PROGRAM MAIN
VAR
	MisMotorAxis1 : MIS_Ctrl; //Instance of motor to control
	ProfilePositioni: MIS_ProfilePosition; //instandce of the profilePositioning functione block
	ProfileHomingi: MIS_ProfileHoming; //Instance of the Homing profile function block
	MISenableMotori: MIS_EnableMotor;
	ChangeMode: MIS_ChangeDSP402Mode;
	ProfileVelocityi: MIS_ProfileVelocity;

	//Test variables
	bModeactive: BOOL;
	eCommandLocal: ECOMMAND;
	diTargetVelocity : DINT := 75;
	rPos1 : REAL := 10;
	rpos2 : REAL := -10; 
END_VAR

VAR_INPUT
	iState : INT ; //State of main function
END_VAR

//wNodeID CANopen node adress of motor
//ADSNetID Adress of the CANopen adapter. Get the ADS net id from the CANopen master adapter, In this example is used an EL6751 adapter
//lrUnitConversion Counts pr unit. This sample uses counts Pr revolution as Convertion factor.
MisMotorAxis1(wNode := 5,ADSNetID := '5.80.217.236.3.1',lrUnitConversion := 409600);


CASE iState OF
0:
	//Reset function blocks
	ProfilePositioni(eCmd := eCommand.Reset,stMisMotorLocal := MisMotorAxis1.stMisMotori);
	ProfileHomingi(eCmd := eCommand.Reset,stMisMotorLocal := MisMotorAxis1.stMisMotori);
	ProfileVelocityi(eCmd := eCommand.Reset,stMisMotorLocal := MisMotorAxis1.stMisMotori);
	ChangeMode(eCmd := eCommand.Reset,stMisMotorLocal := MisMotorAxis1.stMisMotori);

	
	// Set iState to a value to try the function block.
	//
	// 10 Profile postition mode
	// 50 Velocity mode
	// 70 Homing mode
	// 100 Enable motor
	// 110 Disable motor 
	

/////////////////////////////////////////////////////////////////////////////////////////////////////////////////////////////	
10: //Test Profile position
	ChangeMode(eCmd := eCommand.Run,siModeOfOperation := 1,stMisMotorLocal := MisMotorAxis1.stMisMotori);
	IF ChangeMode.eStat = eStatus.Done THEN
		ChangeMode(eCmd := eCommand.Reset,stMisMotorLocal := MisMotorAxis1.stMisMotori);
		bModeactive := TRUE;
		iState := iState + 1;
		eCommandLocal := eCommand.Run;		
	END_IF
11:
	ProfilePositioni(eCmd := eCommand.Reset,rVelocityRpm := 100, rAccellRpms := 100, lrTargetPos := rPos1,stMisMotorLocal := MisMotorAxis1.stMisMotori);
	//iState := 20;  //Sequntial profiles 
	iState := 30; //Overlapping profiles
	
		
//Alternating between 2 positions. Waiting for position reached before next profile prepared
//This allow aborting with quickstop by appliyng the Command stop
20: //Alternate between 2 positions. Wait for position reached 
	IF NOT bModeactive THEN eCommandLocal := eCommand.Stop; END_IF; //Force stop
	ProfilePositioni(eCmd := eCommandLocal,stMisMotorLocal := MisMotorAxis1.stMisMotori);
	IF ProfilePositioni.eStat = eStatus.Done THEN //Wait for position reached
		iState := iState + 1;
	END_IF
	
21:
	IF ProfilePositioni.lrTargetPos <> rPos1 THEN 
		ProfilePositioni(eCmd := eCommand.Reset,rVelocityRpm := 100, rAccellRpms := 100, lrTargetPos := rPos1,stMisMotorLocal := MisMotorAxis1.stMisMotori);
	ELSE
		ProfilePositioni(eCmd := eCommand.Reset,rVelocityRpm := 200, rAccellRpms := 50, lrTargetPos := rPos2,stMisMotorLocal := MisMotorAxis1.stMisMotori);
	END_IF
	iState := iState + 1;

22:	
	IF bModeactive THEN
		iState := 20;
	END_IF;
	

//Laternating between positions. Next position prepared before previus completed.
//Use the bChangeEmidiatly if new Targetdata should be used before position is reached
30:
	IF NOT bModeactive THEN eCommandLocal := eCommand.Stop; END_IF; //Force stop
	ProfilePositioni(eCmd := eCommandLocal,stMisMotorLocal := MisMotorAxis1.stMisMotori);
	IF ProfilePositioni.eStat = eStatus.CmdOk THEN //Wait for command completed
		iState := iState + 1;
	END_IF
	
31: //Preare next commands
	IF ProfilePositioni.lrTargetPos <> rPos1 THEN 
		ProfilePositioni(eCmd := eCommand.Reset,rVelocityRpm := 100, rAccellRpms := 100, lrTargetPos := rPos1,stMisMotorLocal := MisMotorAxis1.stMisMotori);
	ELSE
		ProfilePositioni(eCmd := eCommand.Reset,rVelocityRpm := 200, rAccellRpms := 50, lrTargetPos := rPos2,stMisMotorLocal := MisMotorAxis1.stMisMotori);
	END_IF
	iState := iState + 1;

32:	
	IF bModeactive THEN
		iState := 30;
	END_IF;
	
	



/////////////////////////////////////////////////////////////////////////////////////////////////////////////////////////////
50: //test profile velocity mode 
	ChangeMode(eCmd := eCommand.Run,siModeOfOperation := 3,stMisMotorLocal := MisMotorAxis1.stMisMotori);
	IF ChangeMode.eStat = eStatus.Done THEN
		ChangeMode(eCmd := eCommand.Reset,stMisMotorLocal := MisMotorAxis1.stMisMotori);
		iState := iState + 1;
	END_IF
	
51:
	ProfileVelocityi(eCmd := eCommand.Run,rVelocityRpm := ANY_TO_REAL(diTargetVelocity),rAccellRpms := 125,stMisMotorLocal := MisMotorAxis1.stMisMotori);
	
		
	
/////////////////////////////////////////////////////////////////////////////////////////////////////////////////////////////
70: //Test profile homing mode
	ChangeMode(eCmd := eCommand.Run,siModeOfOperation := 6,stMisMotorLocal := MisMotorAxis1.stMisMotori);
	IF ChangeMode.eStat = eStatus.Done THEN
		ChangeMode(eCmd := eCommand.Reset,stMisMotorLocal := MisMotorAxis1.stMisMotori);
		iState := iState + 1;
	END_IF

71:
	ProfileHomingi(eCmd := eCommand.Run,iHomingMode := 3,rVelocityRpmSearch := 100,rVelocityRpmCrawl := 25,rAccellRpms := 100,lrHomePos := 20.0, stMisMotorLocal := MisMotorAxis1.stMisMotori);
	IF ProfileHomingi.eStat = eStatus.Done OR ProfileHomingi.eStat = eStatus.Error THEN
		ProfileHomingi(eCmd := eCommand.Reset,stMisMotorLocal := MisMotorAxis1.stMisMotori);
		iState := iState + 1;
	END_IF;

/////////////////////////////////////////////////////////////////////////////////////////////////////////////////////////////
100: //Enable motor
	MISenableMotori(eCmd := eCommand.Run,bEnable := TRUE,stMisMotorLocal := MisMotorAxis1.stMisMotori);
	IF MISenableMotori.eStat = eStatus.Done OR MISenableMotori.eStat = eStatus.Error THEN
		 MISenableMotori(eCmd := eCommand.Reset,stMisMotorLocal := MisMotorAxis1.stMisMotori);
		 iState := iState + 1;
	END_IF;
		 
/////////////////////////////////////////////////////////////////////////////////////////////////////////////////////////////
110://Disable motor
	MISenableMotori(eCmd := eCommand.Run,bEnable := FALSE,stMisMotorLocal := MisMotorAxis1.stMisMotori);
	IF MISenableMotori.eStat = eStatus.Done OR MISenableMotori.eStat = eStatus.Error THEN
		 MISenableMotori(eCmd := eCommand.Reset,stMisMotorLocal := MisMotorAxis1.stMisMotori);
		 iState := iState + 1;
	END_IF;
		
		
END_CASE

END_PROGRAM
